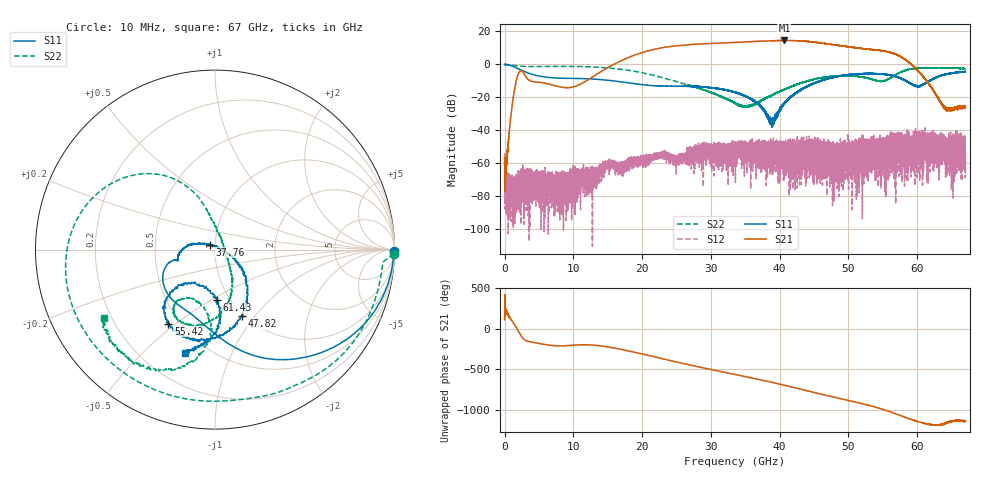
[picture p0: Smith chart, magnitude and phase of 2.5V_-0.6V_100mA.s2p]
! MARKI MICROWAVE INC.
! Date:  10/21/2020
! Model Number:  AMM-7210CH
! Description:  2-port Small Signal S-parameter data for AMM-7210CH
! Frequency Range:  10 MHz to 67 GHz
! Port Configuration:  PORT 1: Input
!  PORT 2: Output
! Bias Condition: Vd = +2.5V, Vg = -0.6V
! AMM-7210CH s2p files are only valid for small signal conditions (below -10 dBm input power)
# Hz S  dB  R 50
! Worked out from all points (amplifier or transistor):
!   20001 points, 10 MHz to 67 GHz, reference 50 ohm
!   highest |S21| = 14.4 dB at 40.69 GHz (marker M1)
!   |S21| within 3 dB of that: 25.55 GHz to 48.48 GHz (22.93 GHz wide, 62 % of centre)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
!   unconditionally stable (mu >= 1): 16.68217 MHz to 16.71573 MHz; 23.36 MHz to end of sweep
!   at 11.17 GHz: K = 1308.35, MAG = -5.8 dB, |S12| = -68.6 dB
!   at 33.51 GHz: K = 54.09, MAG = 13.3 dB, |S12| = -54.1 dB
!   at 67 GHz: K = 1433.66, MAG = -21.3 dB, |S12| = -53.1 dB
!   S11 on the Smith chart (normalised r, x): 10 MHz: open; 37.76 GHz: 0.94, +0.05; 47.82 GHz: 0.98, -0.86; 55.42 GHz: 0.43, -0.47; 61.43 GHz: 0.87, -0.53; 67 GHz: 0.39, -0.67
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1e7  -0.01 -0.6  -57.42 108.8  -55.58 -143.4  -0.01 -1.4
2.22067e9  -3.22 -62.4  -4.30 -61.2  -71.12 7.7  -1.15 -61.5
1.117723e10  -8.76 -133.2  -11.81 161.8  -72.05 -142.6  -1.47 -169.4
1.698862e10  -10.78 -161.1  2.15 105.3  -64.19 133.3  -3.17 148.9
1.988928e10  -12.39 -165.4  6.89 51.9  -59.35 127.0  -5.13 130.2
2.234112e10  -13.27 -164.1  9.50 3.1  -54.93 102.4  -7.51 117.1
2.471256e10  -13.46 -164.5  11.04 -43.8  -56.49 84.6  -10.21 107.8
2.777401e10  -13.51 -169.7  12.11 -101.5  -51.64 97.0  -14.00 99.4
3.088234e10  -14.72 179.8  12.73 -156.9  -50.89 39.0  -18.52 86.1
3.3505e10  -17.02 168.0  13.23 157.3  -54.12 58.3  -23.80 57.3
3.58798e10  -21.30 157.2  13.68 115.6  -52.36 -33.8  -25.18 -6.4
3.775552e10  -28.02 135.6  14.02 81.0  -52.52 -54.4  -21.25 -36.1
4.069303e10  -23.61 -13.4  14.41 24.4  -52.95 -58.4  -15.25 -56.8
4.258214e10  -17.06 -29.9  14.22 -13.8  -51.60 -115.2  -12.18 -68.6
4.467223e10  -12.23 -45.1  13.58 -57.1  -65.39 -4.2  -9.53 -80.7
4.781741e10  -7.98 -68.0  11.79 -119.8  -50.76 160.5  -7.28 -102.1
5.128415e10  -5.92 -94.3  9.90 172.5  -51.34 71.6  -7.38 -122.7
5.541743e10  -6.25 -122.2  7.81 77.6  -80.88 -80.2  -9.97 -102.4
5.583612e10  -6.58 -125.5  7.42 65.5  -47.77 -15.8  -9.01 -98.2
5.86162e10  -10.84 -135.3  1.63 -20.0  -44.21 145.2  -3.46 -106.0
6.143313e10  -10.99 -88.1  -10.62 -90.9  -49.89 155.0  -2.20 -126.5
6.7e10  -4.63 -106.7  -26.47 -57.3  -53.12 175.5  -2.66 -148.4
